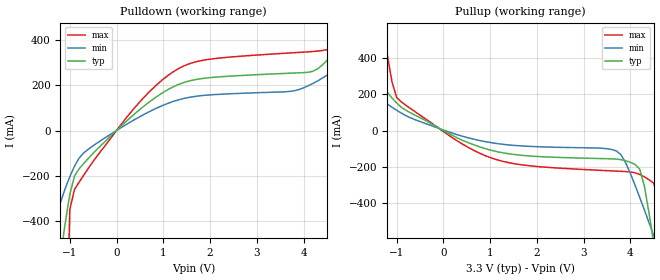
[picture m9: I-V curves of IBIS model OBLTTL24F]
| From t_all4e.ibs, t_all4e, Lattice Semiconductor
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|   OBLTTL24F
[Model]   OBLTTL24F
Model_type   Output
Polarity   Non-Inverting
C_comp   2pF   2pF   2pF
[Temperature Range]   25.0000   125.0000   -40.0000
[Voltage Range]   3.3000V   3.0000V   3.6000V
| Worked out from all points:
|   slope of the pulldown table from 0 to 0.495 V, typ, clamps not added: 5.38 ohm
|   slope of the pullup table from 0 to 0.495 V, typ, clamps not added: 7.79 ohm
[Pulldown]
|voltage   I(typ)   I(min)   I(max)
-3.3V     -4.498A    -1.846A    -40.63A
-1.4V     -903mA     -451.1mA   -5.99A
-1.1V     -408.8mA   -256.1mA   -1.157A
-900mV    -200.2mA   -157.4mA   -259.4mA
-800mV    -168mA     -121mA     -227.2mA
500mV     92.94mA    61.11mA    126.4mA
1.4V      208.4mA    139.1mA    280.1mA
3.9V      253.8mA    180.1mA    343.6mA
4.4V      287.4mA    230.2mA    351.9mA
5.1V      466.4mA    336.6mA    1.051A
5.7V      655mA      446.7mA    2.093A
6.6V      955.9mA    625.4mA    3.709A
[Pullup]
|voltage   I(typ)   I(min)   I(max)
-3.3V     916.1mA    558.1mA    4.19A
-2.3V     572.9mA    351.3mA    2.362A
-1.3V     243mA      162.7mA    581.2mA
-1V       151.9mA    112mA      182.5mA
-500mV    71.07mA    49.53mA    85.15mA
1.2V      -119.4mA   -73.7mA    -165.3mA
3.7V      -157.6mA   -112.4mA   -224mA
4.2V      -213.3mA   -369.2mA   -242.4mA
4.5V      -625.2mA   -580.3mA   -291.2mA
4.6V      -801.4mA   -652.2mA   -378.6mA
4.7V      -981.9mA   -724.6mA   -1.215A
6.6V      -4.576A    -2.132A    -35.2A
[Ramp]
| variable   typ   min   max
dV/dt_r   1.7016/0.2402ns   1.3987/0.4399ns   1.9654/0.1226ns
dV/dt_f   1.7950/0.1991ns   1.5459/0.4478ns   2.0177/0.1041ns
